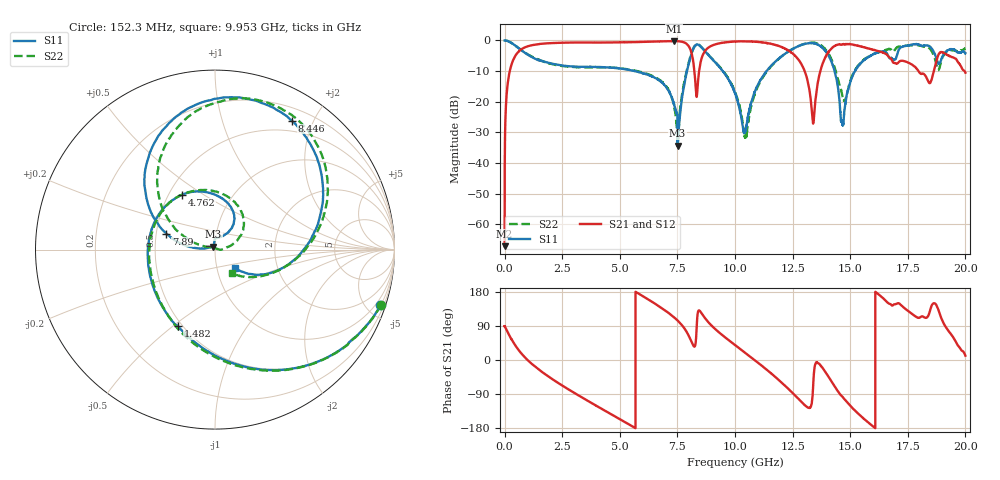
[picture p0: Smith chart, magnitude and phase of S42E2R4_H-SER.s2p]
! Created Wed Nov 25 21:40:35 2020
# khz S ma R 50
! 2 Port Network Data from SP1.SP block
! freq  magS11  angS11  magS21  angS21  magS12  angS12  magS22  angS22
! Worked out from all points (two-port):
!   20001 points, 300 kHz to 20 GHz, reference 50 ohm
!   highest |S21| = -0.22 dB at 7.347 GHz (marker M1); lowest = -67.2 dB at 300 kHz (marker M2)
!   |S21| within 3 dB of the highest: 670.7 MHz to 8.076 GHz (7.406 GHz wide, 169 % of centre); 8.722 GHz to 12.31 GHz (3.587 GHz wide, 34.1 % of centre)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
!   lowest |S11| = -34.4 dB at 7.507 GHz (marker M3), VSWR 1.04, Z = 49 + j1.62 ohm
!   |S11| at or under -10 dB: 5.644 GHz to 7.915 GHz (2.271 GHz wide, 33.5 % of centre); 9.47 GHz to 11.37 GHz (1.901 GHz wide, 18.2 % of centre); 14.32 GHz to 15.21 GHz (884.9 MHz wide, 5.99 % of centre)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
!   |S22| runs from -34.5 to 0.0 dB; largest |S21 - S12| = 0.015
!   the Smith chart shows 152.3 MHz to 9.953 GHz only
!   S11 on the Smith chart (normalised r, x): 152.3 MHz: 0.55, -6.08; 1.482 GHz: 0.47, -0.52; 4.762 GHz: 0.58, +0.41; 7.89 GHz: 0.57, +0.11; 8.446 GHz: 0.36, +1.70; 9.953 GHz: 1.22, -0.26
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300  0.9991 -0.3  0.0004386 88.8  0.0004928 91.4  1 -0.3
152300  0.9719 -18.5  0.2209 71.1  0.2224 71.1  0.9727 -18.5
1482300  0.4741 -115.9  0.8688 -25.1  0.869 -25.2  0.4874 -115.0
3334300  0.3714 169.3  0.9262 -97.9  0.9256 -97.9  0.3653 174.3
4762300  0.3562 121.1  0.9285 -147.7  0.9282 -147.7  0.3589 123.3
6667300  0.2285 63.2  0.9627 143.1  0.9619 143.1  0.2346 47.4
7347300  0.09282 58.0  0.9755 112.9  0.9745 113.0  0.08897 13.6
7507300  0.01915 120.1  0.9705 104.2  0.9708 104.4  0.02153 140.6
7890300  0.2856 161.9  0.8861 75.3  0.8871 75.2  0.3021 147.4
8446300  0.8364 59.3  0.326 130.8  0.3254 130.6  0.8452 53.1
9953300  0.1526 -42.4  0.9589 41.7  0.961 41.8  0.1608 -55.0
1.00003e7  0.1379 -43.3  0.9611 39.5  0.9618 39.6  0.1452 -58.3
1.04603e7  0.03508 40.4  0.967 18.2  0.969 18.3  0.02614 -168.6
1.19633e7  0.5285 33.8  0.7953 -56.3  0.7993 -55.9  0.5265 29.7
1.33343e7  0.9046 -53.9  0.07101 -113.7  0.072 -114.0  0.9172 -61.8
1.40493e7  0.5749 -123.8  0.6416 -43.3  0.638 -43.5  0.6134 -122.7
1.46593e7  0.04303 -105.7  0.8596 -96.6  0.8615 -96.4  0.1237 -124.2
1.53273e7  0.3692 -55.7  0.8205 -140.4  0.8266 -140.9  0.379 -62.3
1.66673e7  0.5366 -122.0  0.545 149.6  0.5339 149.5  0.7252 -121.0
1.84423e7  0.801 174.8  0.2009 125.5  0.2014 126.0  0.7483 157.3
1.90593e7  0.5928 -177.4  0.6297 96.3  0.631 96.2  0.5787 177.7
2e7  0.6147 150.0  0.2972 11.3  0.2986 12.0  0.7391 133.2
